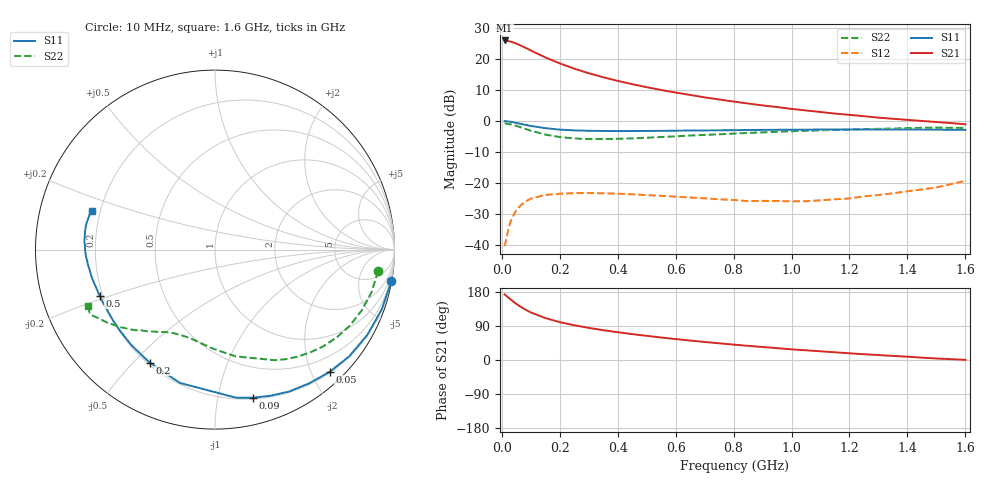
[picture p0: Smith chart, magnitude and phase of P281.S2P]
! Date: Tue Aug 08 16:27:01 1995
# MHZ  S  MA  R  50.0000
!  POLYFET RF DEVICES
!  P281
!  S PARAMETERS
!  VDS=28V, IDQ=200mA
!FREQ  S11MAG S11ANG S21MAG S21ANG S12MAG S12ANG S22MAG S22ANG
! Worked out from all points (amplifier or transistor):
!   40 points, 10 MHz to 1.6 GHz, reference 50 ohm
!   highest |S21| = 26.0 dB at 10 MHz (marker M1)
!   |S21| within 3 dB of that: start of sweep to 95.54 MHz
!   unconditionally stable (mu >= 1): 823.2 MHz to 1.241 GHz
!   at 70 MHz: K = 0.07, MSG = 25.5 dB, |S12| = -26.8 dB
!   at 650 MHz: K = 0.76, MSG = 16.5 dB, |S12| = -24.7 dB
!   at 1.6 GHz: K = 0.56, MSG = 9.1 dB, |S12| = -19.3 dB
!   S11 on the Smith chart (normalised r, x): 10 MHz: 0, -11; 50 MHz: 0.22, -2.29; 90 MHz: 0.21, -1.27; 200 MHz: 0.21, -0.56; 500 MHz: 0.19, -0.19; 1.6 GHz: 0.17, +0.15
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10  0.9983 -10.1  19.92 173.3  0.0096 77.5  0.9165 -7.5
20  0.9869 -19.8  19.6 166.6  0.01559 77.2  0.904 -15.2
30  0.9726 -29.4  19.11 160.2  0.02375 71.2  0.8853 -22.4
40  0.9557 -38.5  18.47 154.1  0.02969 66.2  0.8629 -29.3
50  0.9337 -46.9  17.75 148.4  0.03639 60.3  0.8366 -35.7
60  0.9111 -54.9  16.94 143.1  0.04111 55.9  0.8091 -41.8
70  0.892 -62.5  16.13 138.2  0.04568 52.0  0.78 -47.3
80  0.871 -69.2  15.33 133.7  0.04938 47.6  0.7525 -52.5
90  0.8516 -75.6  14.55 129.6  0.05296 44.2  0.7267 -57.2
100  0.8341 -81.8  13.76 125.8  0.05606 40.9  0.7006 -61.6
150  0.7681 -104.7  10.65 110.7  0.06428 28.5  0.6054 -79.2
200  0.7271 -120.1  8.512 100.0  0.06723 20.1  0.5525 -91.1
250  0.7075 -131.2  7.001 91.7  0.06875 14.2  0.5247 -99.6
300  0.6964 -139.4  5.908 84.8  0.06911 10.1  0.5121 -106.0
400  0.6894 -150.5  4.442 73.4  0.06736 4.6  0.5172 -115.0
500  0.6924 -158.3  3.516 63.8  0.06382 1.4  0.5379 -121.4
550  0.6941 -161.3  3.168 59.4  0.06225 0.7  0.553 -123.8
700  0.7056 -169.1  2.411 47.6  0.05672 1.3  0.5976 -130.6
850  0.7159 -175.2  1.918 37.4  0.05102 6.8  0.6433 -136.1
1100  0.7296 176.3  1.399 22.9  0.05267 22.5  0.7064 -143.9
1350  0.7313 169.2  1.088 10.7  0.06834 36.5  0.7564 -149.8
1600  0.7204 162.6  0.8875 0.4  0.1086 33.9  0.7729 -156.0
